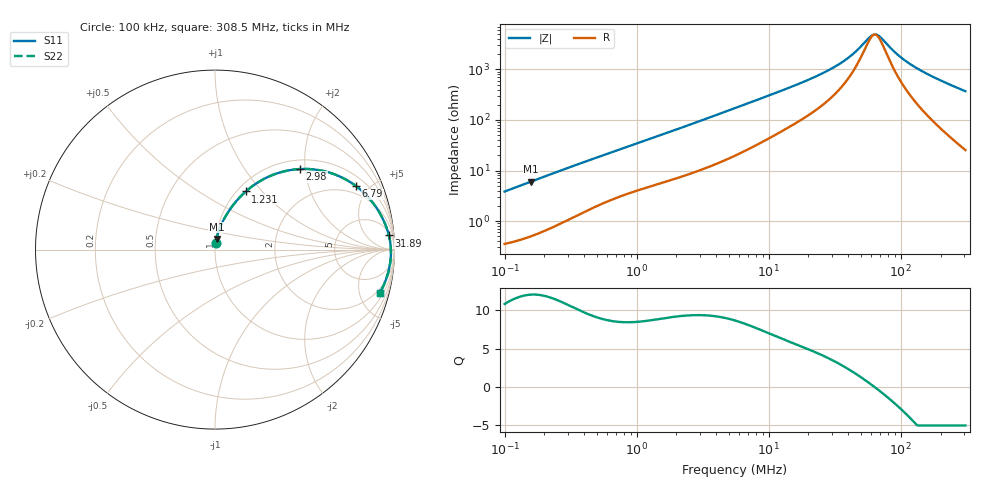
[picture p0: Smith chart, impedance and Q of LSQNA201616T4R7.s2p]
! LSQNA201616T4R7  S-PARAMETER MODEL  ( General Type )
! Model Generated by TAIYO YUDEN Corporation (http://www.ty-top.com)
! Version 2.0
! TAIYO YUDEN Control No. 100810NF25SB-FKC
! Copyright(c) 2007 TAIYO YUDEN CO.,LTD. All Rights Reserved.
! Product Description (link to TY-COMPAS)
! https://ds.yuden.co.jp/TYCOMPAS/or/detail?pn=LSQNA201616T4R7M&u=M
! Products Name : Inductors
! Characteristics :
!  Inductance : 4.7 uH , SRF(min) : 45 MHz , DC Resistance(max) : 0.325 Ohm
!  Rated Current : Saturation :340 mA , Temp Rise : 740 mA (40 degC)
!  Case Size : 2.0 x 1.6 / 0.079 x 0.063 [mm/inch] , Thickness : 1.6 / 0.063 [mm/inch]
!  (Conditions: Temperature = 25 degC , DC Bias Current/Voltage = 0A / 0V)
! External Node Assignments :
!  1  o---GGG---o  2
! GND o---------o GND
! Frequency Range : 0.1MHz  -  308.54851MHz  [ 402 STEP ]
# MHz S RI R 50
! Freq[MHz].  S11 Real  S11 Imag  S21 Real  S21 Imag  S12 Real  S12 Imag  S22 Real  S22 Imag
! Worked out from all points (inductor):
!   401 points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, 100 kHz to 308.5 MHz, reference 50 ohm
!   read as one part in series: L = 6.06 uH near 104.1 kHz
!   highest Q = 12.1 at 158.7 kHz (marker M1), where L = 6.04 uH
!   self-resonance near 63.49 MHz
!   S11 on the Smith chart (normalised r, x): 100 kHz: 1.01, +0.08; 1.231 MHz: 1.09, +0.82; 2.98 MHz: 1.20, +1.88; 6.79 MHz: 1.51, +4.14; 31.89 MHz: 8, +22; 308.5 MHz: 1.51, -7.40
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0.1  0.00495 0.0379  0.995 -0.0379  0.995 -0.0379  0.00495 0.0379
0.158722  0.00854 0.0595  0.9915 -0.0595  0.9915 -0.0595  0.00854 0.0595
0.384115  0.0328 0.1345  0.9672 -0.1345  0.9672 -0.1345  0.0328 0.1345
0.730479  0.0847 0.2258  0.9153 -0.2258  0.9153 -0.2258  0.0847 0.2258
1.231441  0.1716 0.3238  0.8284 -0.3238  0.8284 -0.3238  0.1716 0.3238
1.475446  0.2167 0.3595  0.7833 -0.3595  0.7833 -0.3595  0.2167 0.3595
2.980157  0.4744 0.4489  0.5256 -0.4489  0.5256 -0.4489  0.4744 0.4489
4.027994  0.603 0.4381  0.397 -0.4381  0.397 -0.4381  0.603 0.4381
5.667415  0.7314 0.3892  0.2686 -0.3892  0.2686 -0.3892  0.7314 0.3892
6.790391  0.7864 0.3533  0.2136 -0.3533  0.2136 -0.3533  0.7864 0.3533
11.2196  0.8899 0.2469  0.1101 -0.2469  0.1101 -0.2469  0.8899 0.2469
21.33651  0.9513 0.134  0.0487 -0.134  0.0487 -0.134  0.9513 0.134
31.88523  0.969 0.0791  0.031 -0.0791  0.031 -0.0791  0.969 0.0791
42.23922  0.9758 0.0454  0.0242 -0.0454  0.0242 -0.0454  0.9758 0.0454
57.09072  0.9795 0.0117  0.0205 -0.0117  0.0205 -0.0117  0.9795 0.0117
61.86696  0.98 0.00285  0.02 -0.00285  0.02 -0.00285  0.98 0.00285
68.40302  0.9803 -0.00823  0.0197 0.00823  0.0197 0.00823  0.9803 -0.00823
81.95682  0.9801 -0.0285  0.0199 0.0285  0.0199 0.0285  0.9801 -0.0285
102.2213  0.9783 -0.0547  0.0217 0.0547  0.0217 0.0547  0.9783 -0.0547
135.4153  0.973 -0.0917  0.027 0.0917  0.027 0.0917  0.973 -0.0917
198.3402  0.9576 -0.1523  0.0424 0.1523  0.0424 0.1523  0.9576 -0.1523
308.5485  0.9178 -0.2425  0.0822 0.2425  0.0822 0.2425  0.9178 -0.2425
